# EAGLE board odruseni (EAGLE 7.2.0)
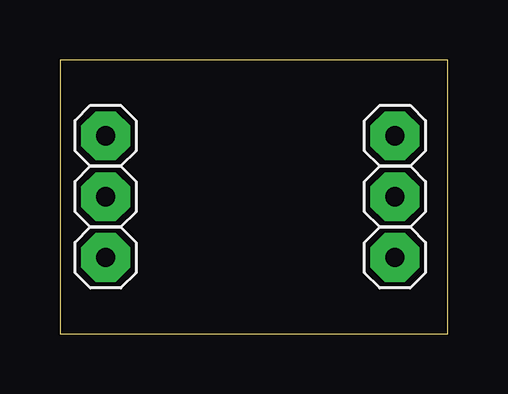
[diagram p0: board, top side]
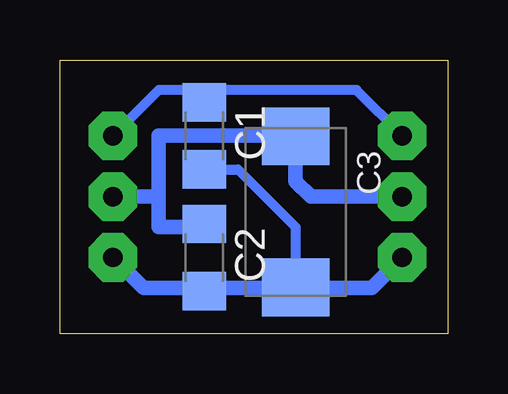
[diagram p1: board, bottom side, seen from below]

Size 16.18 x 11.42 mm. Coordinates in mm from the lower left corner, seen from the top.
Outline: 0,0 16.18,0 16.18,11.42 0,11.42 0,0
Copper layers (1*16): Top 0.035mm / dielectric 1.5mm / Bottom 0.035mm
Design rules "default": minimum track width 10mil, minimum drill 24mil, track to track 8mil, track to pad 8mil, pad to pad 8mil, via to via 8mil, smd to smd 8mil, copper to edge 40mil, drill to drill 8mil, minimum pad ring 10mil, minimum via ring 8mil, stop-mask expansion 4mil, vias tented up to drill 0mil, thermal gap 10mil

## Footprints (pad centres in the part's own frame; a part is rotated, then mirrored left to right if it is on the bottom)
C1206 = smd 1.6 x 1.8: 1 -1.4,0; 2 1.4,0
SMC_D = smd 2.4 x 2.8: + -3.15,0; - 3.15,0
CON_1 = drill 0.8 pad 2.032 octagon: P$1 0,0

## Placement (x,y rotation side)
C1  [C1206]  10.16,8.26 270 bottom
C2  [C1206]  10.16,3.17 270 bottom
C3  [SMC_D]  6.35,5.08 270 bottom
U$1  CON_1  [CON_1]  13.97,8.26 0 top
U$2  CON_1  [CON_1]  13.97,5.71 0 top
U$3  CON_1  [CON_1]  1.91,3.17 0 top
U$4  CON_1  [CON_1]  13.97,3.17 0 top
U$5  CON_1  [CON_1]  1.91,5.71 0 top
U$6  CON_1  [CON_1]  1.91,8.26 0 top

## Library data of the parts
C1-C3 = rcl
U$1-U$6 = arduino

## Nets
N$2: C1.2 C2.2 C3.- U$3.P$1 U$4.P$1
N$3: C2.1 C3.+ U$2.P$1 U$5.P$1
N$4: C1.1 U$1.P$1 U$6.P$1

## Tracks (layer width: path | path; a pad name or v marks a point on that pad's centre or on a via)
N$2
  Bottom 0.406: C1.2 8.76,6.86 6.35,4.45 C3.- | 6.35,1.91 6.35,1.77
  Bottom 0.61: U$3.P$1 3.17,1.91 6.35,1.91 10.16,1.91 12.7,1.91 U$4.P$1
  Bottom 0.813: C2.2 10.16,1.91 | C3.- 6.35,1.91
N$3
  Bottom 0.406: 10.29,4.45 C2.1
  Bottom 0.61: U$5.P$1 5.71,5.71 6.35,6.35 C3.+ 6.35,8.26 12.06,8.26 12.06,5.71 | 12.06,5.71 U$2.P$1 | 10.29,4.45 12.06,4.45 12.06,5.71
N$4
  Bottom 0.406: U$6.P$1 3.81,10.16 10.16,10.16 | C1.1 10.16,10.16 | 10.16,10.16 12.06,10.16 U$1.P$1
